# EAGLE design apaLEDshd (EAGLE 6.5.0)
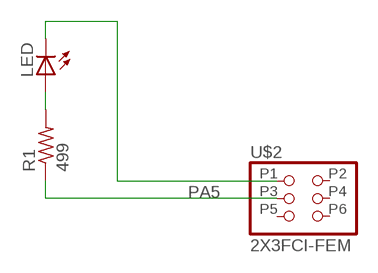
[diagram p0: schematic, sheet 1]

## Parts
LED  LED1206  [1206]
R1  499  RESISTOR1206  [1206]
U$2  2X3FCI-FEM  [2X3FCI-FEM]

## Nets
N$1: LED.1(A) R1.2
N$2: LED.2(C) U$2.P1
PA5: R1.1 U$2.P3
Unconnected: U$2.P2 U$2.P4 U$2.P5 U$2.P6

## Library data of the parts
LED = 01_FAB_Hello:LED
R1 = 01_FAB_Hello:RESISTOR
U$2 = ot:2X3FCI-FEM: 2x3 fci connector It's DEV for using fci 2x3 connector as pin socket on PCB

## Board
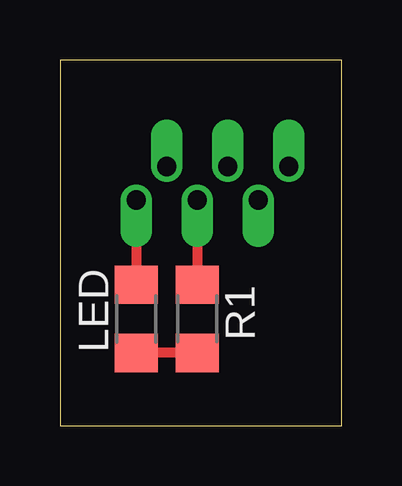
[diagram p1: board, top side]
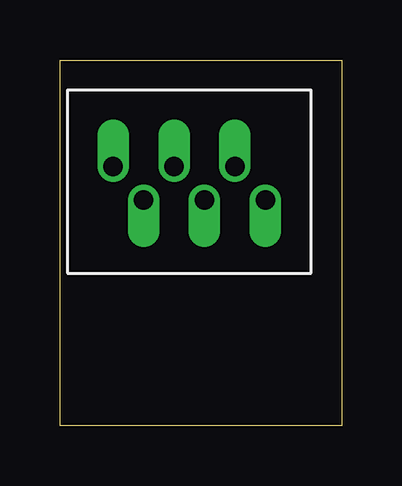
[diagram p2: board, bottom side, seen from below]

Size 11.73 x 15.23 mm. Coordinates in mm from the lower left corner, seen from the top.
Outline: 0,0 11.73,0 11.73,15.23 0,15.23 0,0
Copper layers (1*16): Top 0.035mm / dielectric 1.5mm / Bottom 0.035mm
Design rules "default": minimum track width 10mil, minimum drill 24mil, track to track 8mil, track to pad 8mil, pad to pad 8mil, via to via 8mil, smd to smd 8mil, copper to edge 40mil, drill to drill 8mil, minimum pad ring 10mil, minimum via ring 8mil, stop-mask expansion 4mil, vias tented up to drill 0mil, thermal gap 10mil

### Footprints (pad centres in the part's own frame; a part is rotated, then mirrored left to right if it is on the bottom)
1206 = smd 1.6 x 1.803: 1 -1.422,0; 2 1.422,0
2X3FCI-FEM = drill 0.8 pad 1.27 offset: P1 3.045,8.255; P2 4.445,6.985; P3 3.045,5.715; P4 4.445,4.445; P5 3.045,3.175; P6 4.445,1.905

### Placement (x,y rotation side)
LED  3.17,4.45 90 top
R1  5.71,4.45 270 top
U$2  11.43,6.35 90 top

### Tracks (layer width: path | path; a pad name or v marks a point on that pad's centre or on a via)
N$1
  Top 0.406: R1.2 LED.1
N$2
  Top 0.406: U$2.P1 LED.2
PA5
  Top 0.406: U$2.P3 R1.1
